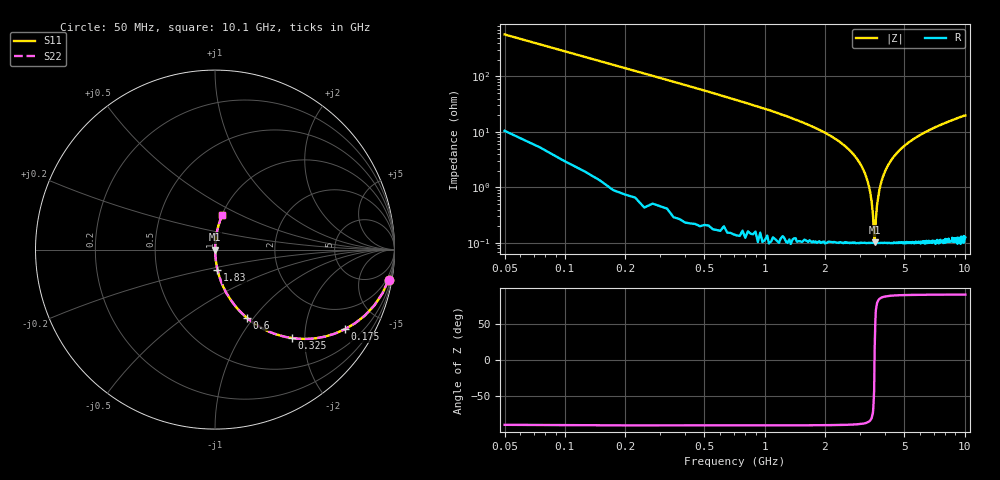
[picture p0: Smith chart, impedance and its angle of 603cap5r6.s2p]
! AVX Thin Film Operation		Date: November 2004
! Description: Accu-P® Series, Thin Film, SMD, RF Capacitor
! Part Number: 06035J5R6ABT
! 50 MHz  -  10.05 GHz
! Serial Measurements
# hz S db R 50
!	S11		S21		S12		S22
!	dB	Phase	dB	Phase	dB	Phase	dB	Phase
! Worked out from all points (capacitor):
!   400 points, 50 MHz to 10.1 GHz, reference 50 ohm
!   read as one part in series: C = 5.6 pF near 100 MHz
!   lowest |Z| = 103 mohm at 3.55 GHz (marker M1)
!   series resonance near 3.546 GHz, so ESL is about 360 pH
!   S11 on the Smith chart (normalised r, x): 50 MHz: 1, -11; 175 MHz: 1.02, -3.24; 325 MHz: 1.01, -1.74; 600 MHz: 1.00, -0.92; 1.83 GHz: 1.00, -0.23; 10.1 GHz: 1.00, +0.40
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5e7  -0.16 -9.9  -15.30 79.0  -15.30 79.0  -0.16 -9.9
1e8  -0.53 -19.3  -9.60 70.1  -9.60 70.1  -0.53 -19.3
1.75e8  -1.43 -31.6  -5.62 58.1  -5.62 58.1  -1.43 -31.6
3.25e8  -3.69 -48.9  -2.45 40.8  -2.45 40.8  -3.69 -48.9
6e8  -7.59 -65.1  -0.85 24.7  -0.85 24.7  -7.59 -65.1
1e9  -11.90 -75.1  -0.30 14.6  -0.30 14.6  -11.90 -75.1
1.73e9  -18.10 -82.4  -0.08 7.2  -0.08 7.2  -18.10 -82.4
1.83e9  -18.90 -83.0  -0.07 6.5  -0.07 6.5  -18.90 -83.0
2.88e9  -29.40 -86.4  -0.01 1.9  -0.01 1.9  -29.40 -86.4
3.18e9  -35.00 -85.7  -0.01 1.0  -0.01 1.0  -35.00 -85.7
3.4e9  -43.40 -81.1  -0.01 0.4  -0.01 0.4  -43.40 -81.1
3.48e9  -49.50 -72.4  -0.01 0.2  -0.01 0.2  -49.50 -72.4
3.55e9  -59.80 13.6  -0.01 -0.0  -0.01 -0.0  -59.80 13.6
3.6e9  -51.50 67.9  -0.01 -0.1  -0.01 -0.1  -51.50 67.9
3.65e9  -46.40 77.7  -0.01 -0.3  -0.01 -0.3  -46.40 77.7
3.75e9  -40.80 83.2  -0.01 -0.5  -0.01 -0.5  -40.80 83.2
3.9e9  -36.30 85.4  -0.01 -0.9  -0.01 -0.9  -36.30 85.4
4.4e9  -29.10 86.4  -0.01 -2.0  -0.01 -2.0  -29.10 86.4
5.08e9  -24.60 85.7  -0.02 -3.4  -0.02 -3.4  -24.60 85.7
6.75e9  -19.20 83.2  -0.06 -6.3  -0.06 -6.3  -19.20 83.2
8.43e9  -16.20 80.7  -0.12 -8.9  -0.12 -8.9  -16.20 80.7
1.01e10  -14.20 78.4  -0.18 -11.2  -0.18 -11.2  -14.20 78.4
